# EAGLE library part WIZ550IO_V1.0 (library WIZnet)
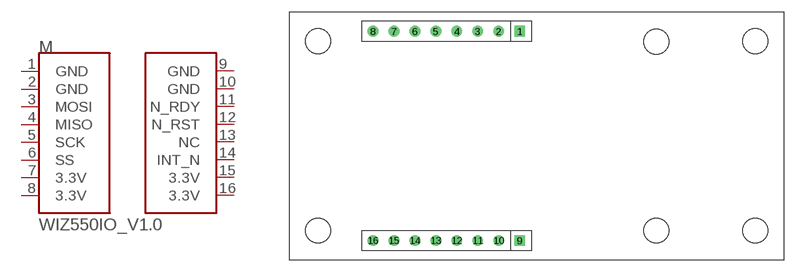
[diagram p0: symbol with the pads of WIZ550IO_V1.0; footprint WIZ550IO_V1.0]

Designator prefix M

## WIZ550IO_V1.0  [WIZ550IO_V1.0]
1  GND  pas
2  GND  pas
3  MOSI  pas
4  MISO  pas
5  SCK  pas
6  SS  pas
7  3.3V  pas
8  3.3V  pas
9  GND  pas
10  GND  pas
11  N_RDY  pas
12  N_RST  pas
13  NC  pas
14  INT_N  pas
15  3.3V  pas
16  3.3V  pas

## Footprint WIZ550IO_V1.0 (pad centres in mm)
drill 0.8 square: 1 -2.06,12.7; 9 -2.06,-12.7
drill 0.8: 2 -4.6,12.7; 3 -7.14,12.7; 4 -9.68,12.7; 5 -12.22,12.7; 6 -14.76,12.7; 7 -17.3,12.7; 8 -19.84,12.7; 10 -4.6,-12.7; 11 -7.14,-12.7; 12 -9.68,-12.7; 13 -12.22,-12.7; 14 -14.76,-12.7; 15 -17.3,-12.7; 16 -19.84,-12.7
hole 3 at -26.5,11.5
hole 3 at -26.5,-11.5
hole 3 at 26.5,11.5
hole 3 at 26.5,-11.5
hole 3 at 14.5,11.43
hole 3 at 14.5,-11.5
